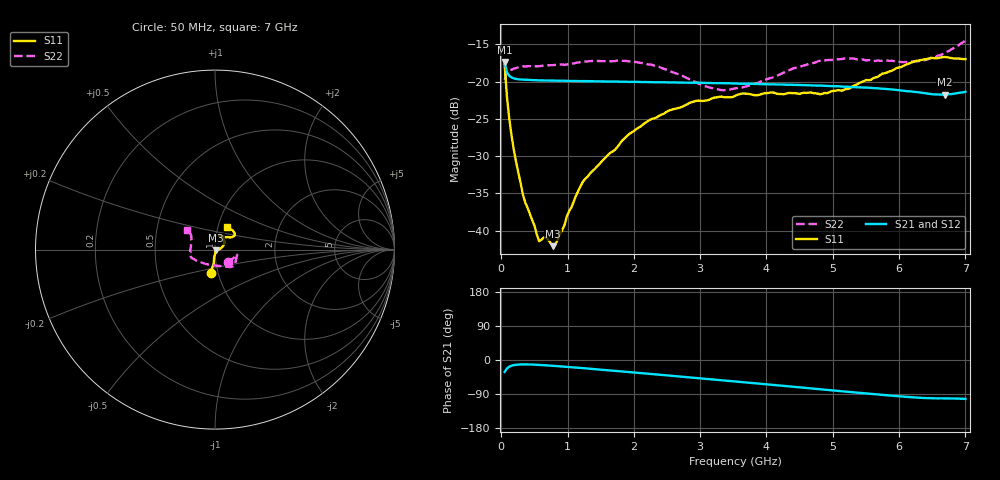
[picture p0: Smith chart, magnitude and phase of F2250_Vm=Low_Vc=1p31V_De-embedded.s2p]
! Integrated Device Technology
! Corporate Headquarters
! 6024 Silver Creek Valley Road
! San Jose, CA 95138  USA
! Phone:  1-408-284-8200
! Toll Free:  1-800-223-1366
! Webpage:  http://www.idt.com/
! Timing and RF Division
! 515 Groton Road, Suite 102
! Westford, MA 01886-6024
! Device:  F2250
! Description: Voltage Variable RF Attenuator
! Frequency:  50.0 -  6000.00 MHz
! Package:  3x3 mm Thin QFN Plastic Package: 16 pin
! Ports:  2 RF, 3 DC
!  Pin  1  = GND
!  Pin  2  = NC
!  Pin  3  = RF1  = Port 1
!  Pin  4  = NC
!  Pin  5  = GND
!  Pin  6  = GND
!  Pin  7  = GND
!  Pin  8  = GND
!  Pin  9  = NC
!  Pin 10  = RF2  = Port 2
!  Pin 11  = NC
!  Pin 12  = GND
!  Pin 13  = GND
!  Pin 14  = VCNTRL
!  Pin 15  = VDD
!  Pin 16  = VMODE
! Vcntrl:  1.310 Volts
! Vmode:  +0.000 Volts
! Vdd:  +3.30  Volts
! Current:  1.192 mA
! Data:  The device was measured on a the F2250 evaluation board which has
!  individual transmission lines to the RF pins.  Data was collected
!  using a calibrated network analyzer.  The evaluation board was
!  de-embedded using a TRL calibration technique.
!  The reference plane is the edge of the package pin.
! Misc:  SN 10
!  Action Tracker AT0258
! Date Measured:  2014-11-26
! Date:  2015-10-15  MJV
! Note:
!  Integrated Device Technology supplies this data as a sample of measured
!  data at the package pin for this product.  Your particular data for this
!  product may vary.
!  Data was taken at 25 degrees C.
!  Integrated Device Technology reserves the right to change this data at anytime.
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# GHz S dB R 50
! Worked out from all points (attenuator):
!   201 points, 50 MHz to 7 GHz, reference 50 ohm
!   highest |S21| = -17.39 dB at 50 MHz (marker M1); lowest = -21.8 dB at 6.687 GHz (marker M2)
!   lowest |S11| = -42.1 dB at 779.8 MHz (marker M3), VSWR 1.02, Z = 50.7 - j0.388 ohm
!   |S11| at or under -10 dB: start of sweep to end of sweep
!   |S22| runs from -21.2 to -14.5 dB; largest |S21 - S12| = 0.00043
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0.05  -17.68 -101.1  -17.39 -31.7  -17.38 -31.6  -19.82 -44.5
0.08475  -21.99 -95.6  -18.76 -22.4  -18.76 -22.4  -18.72 -22.1
0.15425  -27.22 -96.2  -19.44 -15.0  -19.45 -15.0  -18.41 -13.7
0.22375  -30.81 -91.7  -19.65 -12.5  -19.63 -12.5  -18.18 -12.9
0.328  -35.24 -84.8  -19.76 -11.5  -19.74 -11.5  -17.95 -12.9
0.57125  -41.42 -58.2  -19.84 -13.0  -19.84 -13.0  -17.94 -17.5
0.6755  -40.94 -47.7  -19.85 -14.1  -19.86 -14.1  -17.84 -19.9
0.77975  -42.08 -29.1  -19.87 -15.3  -19.87 -15.3  -17.80 -22.6
0.91875  -39.93 -14.8  -19.88 -17.2  -19.89 -17.1  -17.69 -26.5
1.023  -37.39 -16.2  -19.92 -18.5  -19.93 -18.5  -17.64 -28.1
1.2315  -33.42 -1.3  -19.93 -21.5  -19.94 -21.5  -17.33 -32.7
1.9265  -27.06 20.8  -20.05 -31.8  -20.04 -31.8  -17.29 -43.1
2.37825  -24.60 31.6  -20.09 -38.7  -20.09 -38.7  -18.02 -50.8
2.86475  -22.78 46.0  -20.16 -46.3  -20.14 -46.3  -19.80 -66.2
3.14275  -22.42 53.7  -20.19 -50.6  -20.19 -50.6  -20.80 -81.3
3.525  -21.92 64.7  -20.26 -56.7  -20.27 -56.7  -20.92 -107.5
4.7065  -21.55 68.5  -20.52 -75.5  -20.53 -75.5  -17.50 -157.9
5.22775  -20.98 51.7  -20.70 -83.9  -20.71 -83.9  -16.92 -167.1
5.85325  -18.64 36.5  -21.03 -93.7  -21.04 -93.8  -17.22 -180.0
6.33975  -17.09 38.2  -21.49 -100.0  -21.52 -100.0  -17.21 162.4
6.68725  -16.70 46.9  -21.77 -101.3  -21.74 -101.4  -16.11 148.7
7  -16.98 62.7  -21.36 -102.7  -21.36 -102.8  -14.48 145.3
